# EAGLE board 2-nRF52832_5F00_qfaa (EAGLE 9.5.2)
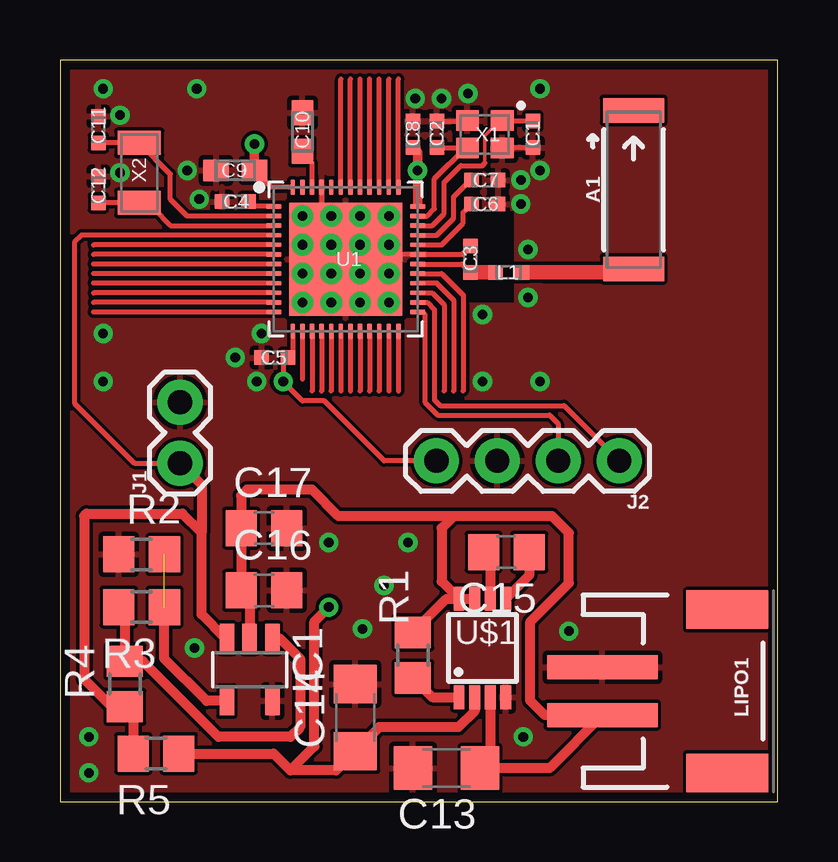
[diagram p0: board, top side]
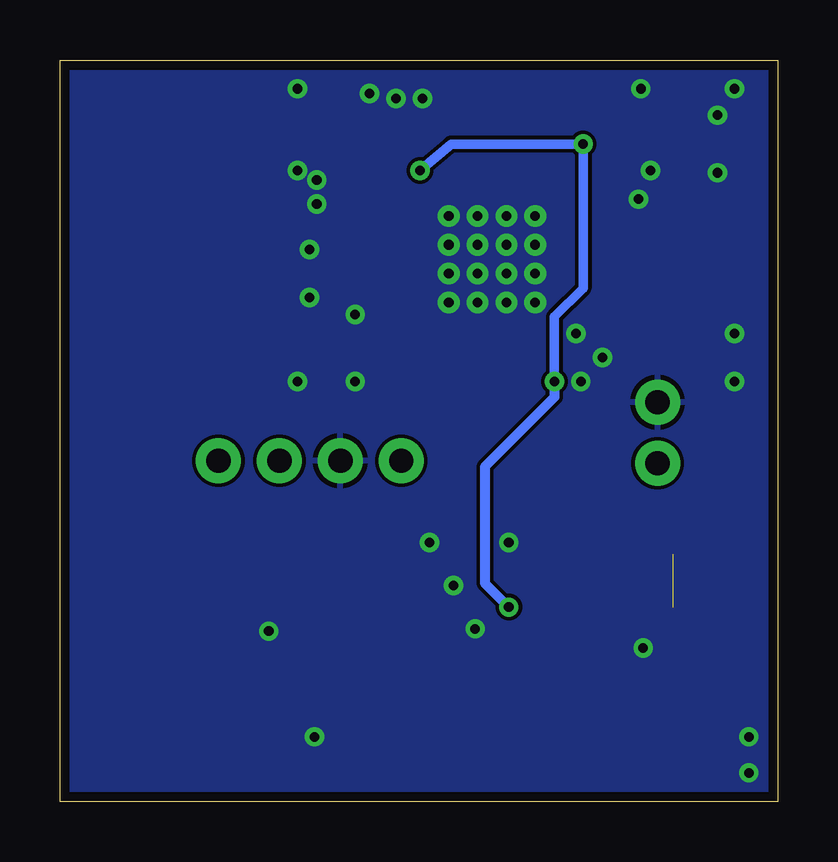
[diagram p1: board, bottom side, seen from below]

Size 29.9 x 30.9 mm. Coordinates in mm from the lower left corner, seen from the top.
Outline: 0,0 29.9,0 29.9,30.9 0,30.9 0,0
Copper layers (1*16): Top 0.035mm / dielectric 1.5mm / Bottom 0.035mm
Design rules "Nordic": minimum track width 0.15mm, minimum drill 0.4mm, track to track 0.15mm, track to pad 0.15mm, pad to pad 0.15mm, via to via 0.15mm, smd to smd 0.15mm, copper to edge 0.4mm, drill to drill 0.4mm, minimum pad ring 10mil, minimum via ring 8mil, stop-mask expansion 4mil, vias tented up to drill 0mil, thermal gap 0.2mm
tRestrict: area 15.3,20.8 to 18.9,24.6

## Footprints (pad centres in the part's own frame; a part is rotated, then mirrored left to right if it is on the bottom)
ANT-2.4GHZ-6.5X2.2MM = smd 1.016 x 2.54: FEED -3.302,0; NC 3.302,0
RESC0402_N = smd 0.6 x 0.6: 1 -0.55,0; 2 0.55,0
RESC0603_N = smd 1.05 x 0.9: 1 -0.8,0; 2 0.8,0
C1206 = smd 1.6 x 1.8: 1 -1.4,0; 2 1.4,0
C0805 = smd 1.3 x 1.5: 1 -0.95,0; 2 0.95,0
SOT23-5 = smd 0.6 x 1.2: 1 -0.95,-1.306; 2 0,-1.306; 3 0.95,-1.306; 4 0.95,1.306; 5 -0.95,1.306
1X02 = drill 1.016 pad 1.88: 1 0,0; 2 2.54,0
1X04 = drill 1.016 pad 1.88: 1 0,0; 2 2.54,0; 3 5.08,0; 4 7.62,0
JST-2-SMD = smd 1 x 4.6: 1 -1,-3.7; 2 1,-3.7 | smd 1.6 x 3.4: NC1 -3.4,1.5; NC2 3.4,1.5
R0805 = smd 1.3 x 1.5: 1 -0.95,0; 2 0.95,0
QFN40P600X600X90-48_N = smd 0.65 x 0.2: 1 -3,2.2; 2 -3,1.8; 3 -3,1.4; 4 -3,1; 5 -3,0.6; 6 -3,0.2; 7 -3,-0.2; 8 -3,-0.6; 9 -3,-1; 10 -3,-1.4; 11 -3,-1.8; 12 -3,-2.2; 25 3,-2.2; 26 3,-1.8; 27 3,-1.4; 28 3,-1; 29 3,-0.6; 30 3,-0.2; 31 3,0.2; 32 3,0.6; 33 3,1; 34 3,1.4; 35 3,1.8; 36 3,2.2 | smd 0.2 x 0.65: 13 -2.2,-3; 14 -1.8,-3; 15 -1.4,-3; 16 -1,-3; 17 -0.6,-3; 18 -0.2,-3; 19 0.2,-3; 20 0.6,-3; 21 1,-3; 22 1.4,-3; 23 1.8,-3; 24 2.2,-3; 37 2.2,3; 38 1.8,3; 39 1.4,3; 40 1,3; 41 0.6,3; 42 0.2,3; 43 -0.2,3; 44 -0.6,3; 45 -1,3; 46 -1.4,3; 47 -1.8,3; 48 -2.2,3 | smd 4.7 x 4.7: PAD 0,0 | drill 0.4: PAD@VIA01 -1.8,1.8; PAD@VIA02 -1.8,0.6; PAD@VIA03 -1.8,-0.6; PAD@VIA04 -1.8,-1.8; PAD@VIA05 -0.6,1.8; PAD@VIA06 -0.6,0.6; PAD@VIA07 -0.6,-0.6; PAD@VIA08 -0.6,-1.8; PAD@VIA09 0.6,1.8; PAD@VIA10 0.6,0.6; PAD@VIA11 0.6,-0.6; PAD@VIA12 0.6,-1.8; PAD@VIA13 1.8,1.8; PAD@VIA14 1.8,0.6; PAD@VIA15 1.8,-0.6; PAD@VIA16 1.8,-1.8
MSOP8 = smd 0.45 x 1: 1 -0.975,-2.05; 2 -0.325,-2.05; 3 0.325,-2.05; 4 0.975,-2.05; 5 0.975,2.05; 6 0.325,2.05; 7 -0.325,2.05; 8 -0.975,2.05
BT-XTAL_2016_N = smd 0.95 x 0.85: 1 -0.725,-0.575; 2 0.725,-0.575; 3 0.725,0.575; 4 -0.725,0.575
XTAL_3215_N = smd 1 x 1.8: 1 -1.25,0; 2 1.25,0

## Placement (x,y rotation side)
A1  2.45GHz  [ANT-2.4GHZ-6.5X2.2MM]  23.9,25.5 90 top
C1  12pF  [RESC0402_N]  19.7,27.8 270 top
C2  12pF  [RESC0402_N]  15.7,27.8 90 top
C3  0.8pF  [RESC0402_N]  17.1,22.6 90 top
C4  100nF  [RESC0402_N]  7.3,25 180 top
C5  100nF  [RESC0402_N]  8.95,18.5 180 top
C6  N.M.  [RESC0402_N]  17.7,24.9 0 top
C7  100pF  [RESC0402_N]  17.7,25.9 0 top
C8  100nF  [RESC0402_N]  14.7,27.8 90 top
C9  4.7µF  [RESC0603_N]  7.3,26.3 180 top
C10  1.0µF  [RESC0603_N]  10.1,27.9 90 top
C11  12pF  [RESC0402_N]  1.6,28 270 top
C12  12pF  [RESC0402_N]  1.6,25.5 270 top
C13  10µF  [C1206]  16.1,1.4 180 top
C14  10µF  [C1206]  12.3,3.5 90 top
C15  1µF  [C0805]  18.6,10.4 180 top
C16  0.1µF  [C0805]  8.5,8.8 0 top
C17  1µF  [C0805]  8.5,11.4 0 top
IC1  MCP601R  [SOT23-5]  7.9,5.5 180 top
J1  [1X02]  5,14.1 90 top
J2  [1X04]  23.3,14.2 180 top
L1  3.9nH  [RESC0402_N]  18.7,22.05 0 top
LIPO1  [JST-2-SMD]  26.3,4.6 270 top
R1  100k  [R0805]  14.7,6.1 90 top
R2  1.8M  [R0805]  3.4,10.3 0 top
R3  1.8M  [R0805]  3.4,8.1 180 top
R4  1.8M  [R0805]  2.7,4.9 90 top
R5  1.8M  [R0805]  4,2 180 top
U1  NRF52832  [QFN40P600X600X90-48_N]  11.9,22.6 0 top
U$1  MCP1252-33X50  [MSOP8]  17.6,6.4 0 top
X1  32MHz  [BT-XTAL_2016_N]  17.7,27.8 180 top
X2  32.768kHz  [XTAL_3215_N]  3.3,26.2 270 top

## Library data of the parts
A1 = SparkFun-RF; PROD_ID: ANT-08187; SF_ID: WRL-00144
C1-C12 L1 U1 X1 X2 = Nordic_nRF
C13-C17 = rcl; SPICEPREFIX: C
IC1 = linear
J1 = CalvEngIO-Connectors
J2 = CalvEngIO-Connectors; PROD_ID: CONN-09696
LIPO1 = CalvEngIO-Connectors; PROD_ID: CONN-11443; SF_ID: PRT-08612
R1-R5 = rcl; SPICEPREFIX: R
U$1 = microchip-mcp125x-xxx

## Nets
ANT: C3.1 L1.1 U1.30
C+: C15.2 U$1.6
C-: C15.1 U$1.5
DEC1: C4.1 U1.1
DEC2: C6.1 U1.32
DEC3: C7.1 U1.33
DEC4: C10.1 U1.46
GND: C1.2 C2.2 C3.2 C4.2 C5.2 C6.2 C7.2 C8.2 C9.2 C10.2 C11.1 C12.1 C13.2 C14.2 C16.2 C17.2 IC1.5 J1.2 J2.3 LIPO1.1 R2.1 U1.31 U1.45 U1.PAD U1.PAD@VIA01 U1.PAD@VIA02 U1.PAD@VIA03 U1.PAD@VIA04 U1.PAD@VIA05 U1.PAD@VIA06 U1.PAD@VIA07 U1.PAD@VIA08 U1.PAD@VIA09 U1.PAD@VIA10 U1.PAD@VIA11 U1.PAD@VIA12 U1.PAD@VIA13 U1.PAD@VIA14 U1.PAD@VIA15 U1.PAD@VIA16 U$1.4 X1.2 X1.4
N$1: IC1.1 R3.2 R4.2
N$3: C2.1 U1.35 X1.3
N$4: R1.1 U$1.1
N$6: IC1.4 R2.2 R3.1
P0.00/XL1: C11.2 U1.2 X2.1
P0.01/XL2: C12.2 U1.3 X2.2
P0.02: IC1.3 J1.1 R4.1 R5.2 U1.4
P0.03: U1.5
P0.04: U1.6
P0.05: U1.7
P0.06: U1.8
P0.07: U1.9
P0.08: U1.10
P0.09: U1.11
P0.10: U1.12
P0.11: U1.14
P0.12: U1.15
P0.13: U1.16
P0.14: U1.17
P0.15: U1.18
P0.16: U1.19
P0.17: U1.20
P0.18/SWO: U1.21
P0.19: U1.22
P0.20: U1.23
P0.21/RESET: U1.24
P0.22: U1.27
P0.23: U1.28
P0.24: U1.29
P0.25: U1.37
P0.26: U1.38
P0.27: U1.39
P0.28: U1.40
P0.29: U1.41
P0.30: U1.42
P0.31: U1.43
RF: A1.FEED L1.2
SWDCLK: J2.2 U1.25
SWDIO: J2.1 U1.26
VDD: C13.1 C16.1 C17.1 IC1.2 LIPO1.2 R1.2 U$1.3 U$1.7 U$1.8
VDD_P3V3: C5.1 C8.1 C9.1 C14.1 J2.4 R5.1 U1.13 U1.36 U1.48 U$1.2
X1: C1.1 U1.34 X1.1

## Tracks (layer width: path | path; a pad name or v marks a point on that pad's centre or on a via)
ANT
  Top 0.2: U1.30 16.75,22.4 C3.1 17.15,22.05
  Top 0.6: L1.1 17.15,22.05
C+
  Top 0.406: C15.2 17.93,10.12 U$1.6
C-
  Top 0.406: C15.1 19.55,9.43 U$1.5
DEC1
  Top 0.2: U1.1 8.05,24.8 C4.1
DEC2
  Top 0.2: U1.32 15.9,23.2 16.8,24.1 16.8,24.55 C6.1
DEC3
  Top 0.2: U1.33 15.7,23.6 16.4,24.3 16.4,25.2 17.05,25.85 C7.1
DEC4
  Top 0.2: U1.46 10.5,26.6 C10.1
GND  (via drill 0.4, 0.4 pad 0.8)
  Top 0.2: 13.75,22.79 U1.31 16.75,22.8 C3.2 | 13.75,22.79 arc-90 U1.PAD@VIA14 | 10.95,24.59 arc90 U1.PAD@VIA05 | U1.PAD@VIA01 10.9,24.4 | 10.9,24.4 U1.PAD@VIA05 | U1.PAD@VIA05 U1.PAD@VIA09 U1.PAD@VIA13 U1.PAD@VIA14 | U1.PAD@VIA02 U1.PAD@VIA06 | U1.PAD@VIA06 U1.PAD@VIA10 U1.PAD@VIA14 | 13.75,22.79 13.75,22.39 arc-90 U1.PAD@VIA15 U1.PAD@VIA16 | U1.PAD@VIA11 U1.PAD@VIA07 U1.PAD@VIA03 U1.PAD@VIA04 U1.PAD@VIA08 | U1.PAD@VIA06 arc90 U1.PAD | U1.45 10.9,24.4 | C1.2 18.45,27.25 X1.4 | C2.2 16.95,28.35 X1.2 | 6.75,26.05 C9.2
  other vias: 2.5,26.2 2.5,28.6 5.3,26.3 14.8,29.3 19.2,25.9 19.2,24.9 5.8,25.1 20,26.3 17,29.5 15.9,29.3 8.2,17.5 8.4,19.5 19.5,21 19.5,23 1.8,29.7 5.7,29.7 20,29.7 17.6,20.3 20,17.5 17.6,17.5 7.3,18.5 1.8,17.5 1.8,19.5 12.6,7.2 11.2,10.8 14.5,10.8 19.3,2.7 21.2,7.1 5.6,6.4 1.2,2.7 1.2,1.2 13.5,9
  pour Top: 0,0 0,30.9 29.9,30.9 29.9,0
  pour Bottom: 0,0 0,30.9 29.9,30.9 29.9,0
N$1
  Top 0.406: R3.2 2.7,7.85 R4.2 3.45,5.85 6.6,2.7 9.6,2.7 10,3.1 10,5.96 9.15,6.81 IC1.1
N$3
  Top 0.2: U1.35 15.3,24.4 15.6,24.7 15.6,25.95 16.9,27.25 | C2.1 16.9,27.25 | 16.9,27.25 16.95,27.25 X1.3
N$4
  Top 0.406: R1.1 15.5,4.35 U$1.1
N$6  (1 unrouted)
  Top 0.406: IC1.4 6.11,4.19 4.35,5.95 R3.1
P0.00/XL1
  Top 0.2: C11.2 X2.1 4.6,26.15 4.6,25.1 5.3,24.4 U1.2
P0.01/XL2
  Top 0.2: C12.2 X2.2 3.55,24.7 3.9,24.7 4.6,24 U1.3
P0.02
  Top 0.2: J1.1 3.1,14.1 0.6,16.6 0.6,23.3 0.9,23.6 U1.4
  Top 0.406: R5.2 3.05,3.6 R4.1 2.15,3.95 1,5.1 1,11.9 1.1,12 5.1,12 5.9,11.2 | IC1.3 6.89,6.81 5.9,7.8 5.9,11.2 | J1.1 5.9,13.2 5.9,11.2
P0.03
  Top 0.2: U1.5 1.4,23.2
P0.04
  Top 0.2: U1.6 1.4,22.8
P0.05
  Top 0.2: U1.7 1.4,22.4
P0.06
  Top 0.2: U1.8 1.4,22
P0.07
  Top 0.2: U1.9 1.4,21.6
P0.08
  Top 0.2: U1.10 1.4,21.2
P0.09
  Top 0.2: U1.11 1.4,20.8
P0.10
  Top 0.2: U1.12 1.4,20.4
P0.11
  Top 0.2: U1.14 10.1,17.6
P0.12
  Top 0.2: U1.15 10.5,17.1
P0.13
  Top 0.2: U1.16 10.9,17.1
P0.14
  Top 0.2: U1.17 11.3,17.1
P0.15
  Top 0.2: U1.18 11.7,17.1
P0.16
  Top 0.2: U1.19 12.1,17.1
P0.17
  Top 0.2: U1.20 12.5,17.1
P0.18/SWO
  Top 0.2: U1.21 12.9,17.1
P0.19
  Top 0.2: U1.22 13.3,17.1
P0.20
  Top 0.2: U1.23 13.7,17.1
P0.21/RESET
  Top 0.2: U1.24 14.1,17.1
P0.22
  Top 0.2: U1.27 15.5,21.2 16,20.7 16,17.1
P0.23
  Top 0.2: U1.28 15.7,21.6 16.4,20.9 16.4,17.1
P0.24
  Top 0.2: U1.29 15.9,22 16.8,21.1 16.8,17.1
P0.25
  Top 0.2: U1.37 14.1,30.1
P0.26
  Top 0.2: U1.38 13.7,30.1
P0.27
  Top 0.2: U1.39 13.3,30.1
P0.28
  Top 0.2: U1.40 12.9,30.1
P0.29
  Top 0.2: U1.41 12.5,30.1
P0.30
  Top 0.2: U1.42 12.1,30.1
P0.31
  Top 0.2: U1.43 11.7,30.1
RF
  Top 0.6: L1.2 20.2,22.05
  Top 0.61: 20.2,22.05 23.75,22.05 A1.FEED
SWDCLK
  Top 0.2: U1.25 15.1,20.4 15.2,20.3 15.2,16.64 15.74,16.1 20.4,16.1 20.76,15.74 J2.2
SWDIO
  Top 0.2: U1.26 15.3,20.8 15.6,20.5 15.6,16.74 15.84,16.5 21,16.5 J2.1
VDD
  Top 0.406: U$1.3 17.93,1.82 C13.1 20.4,1.4 LIPO1.2 20.2,3.6 19.6,4.2 19.6,7.5 21.2,9.1 21.2,11.2 20.5,11.9 16.4,11.9 | U$1.8 U$1.7 | R1.2 16.1,8.45 U$1.8 | 16.4,11.9 15.9,11.4 15.9,9.18 U$1.8 | 16.4,11.9 11.6,11.9 10.5,13 7.8,13 7.55,12.75 C17.1 C16.1 7.9,8.45 IC1.2
VDD_P3V3  (via drill 0.4, 0.4 pad 0.8)
  Top 0.2: U1.48 8.8,25.6 C9.1 | U1.36 14.9,24.9 | U1.13 9.7,18.5 C5.1 9.3,18.5 v9.3,17.5 10.1,16.7 11,16.7 13.5,14.2 J2.4
  Top 0.4: 14.9,24.9 v14.9,26.3 14.9,27.05 C8.1 | v8.1,27.4 C9.1
  Top 0.406: 12.9,2.7 C14.1 | C14.1 11.5,1.3 9.6,1.3 | U$1.2 17.27,3.77 16.6,3.1 13.3,3.1 C14.1 | R5.1 8.9,2 9.6,1.3 | 9.6,1.3 10.6,2.3 10.6,7.5 v11.2,8.1
  Bottom 0.4: v9.3,17.5 9.3,20.2 8.1,21.4 v8.1,27.4 13.6,27.4 v14.9,26.3
  Bottom 0.406: v9.3,17.5 9.3,16.85 12.2,13.95 12.2,9.1 v11.2,8.1
X1
  Top 0.15: 17.7,26.6 17.7,27.75 18.32,28.38 X1.1
  Top 0.2: C1.1 18.45,28.35 X1.1 | U1.34 15.5,24 16,24.5 16,25.8 16.7,26.5 17.6,26.5 17.7,26.6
